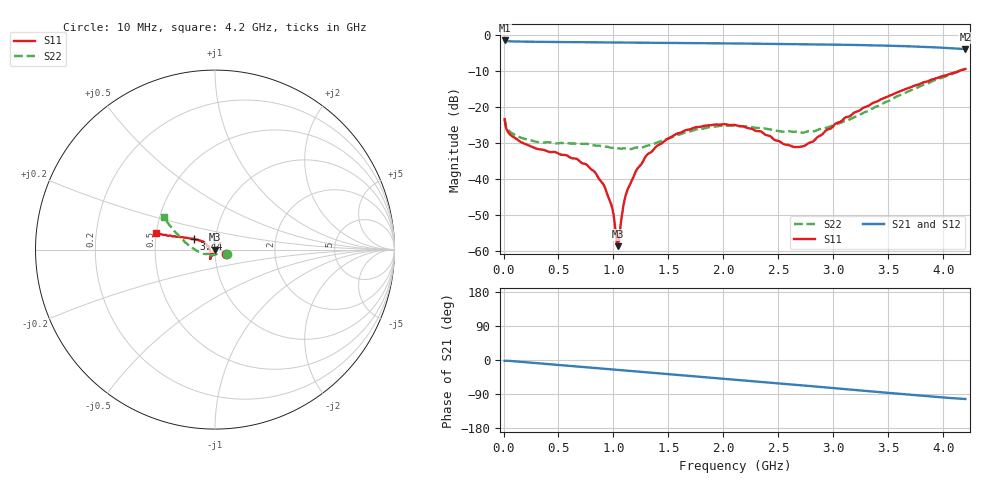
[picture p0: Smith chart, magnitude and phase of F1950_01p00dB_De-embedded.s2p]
! Integrated Device Technology
! Corporate Headquarters
! 6024 Silver Creek Valley Road
! San Jose, CA 95138  USA
! Phone:  1-408-284-8200
! Toll Free:  1-800-223-1366
! Webpage:  http://www.idt.com/
! Timing and RF Division
! 515 Groton Road, Suite 102
! Westford, MA 01886-6024
! Device:  F1950
! Description: 7-bit 0.25 dB Digital Step Attenuator
! Frequency:  150.0 -  4000.00 MHz
! Package:  4x4 mm Thin QFN Plastic Package: 24 pin
! Ports:  2 RF, 12 DC
!  Pin  1  = D0
!  Pin  2  = VDD
!  Pin  3  = Vmode
!  Pin  4  = GND
!  Pin  5  = RF1  =  Port 1
!  Pin  6  = GND
!  Pin  7  = GND
!  Pin  8  = GND
!  Pin  9  = GND
!  Pin 10  = GND
!  Pin 11  = GND
!  Pin 12  = GND
!  Pin 13  = GND
!  Pin 14  = RF2  =  Port 2
!  Pin 15  = GND
!  Pin 16  = LE
!  Pin 17  = CLK
!  Pin 18  = DATE
!  Pin 19  = D6
!  Pin 20  = D5
!  Pin 21  = D4
!  Pin 22  = D3
!  Pin 23  = D2
!  Pin 24  = D1
! State:  4
! Atten State:  1.00 dB
! Voltage:  +5.00 Volts
! Current:  Not Measured mA
! Data:  The device was measured on a the F195X evaluation board which has
!  individual transmission lines to the RF pins.  Data was collected
!  using a calibrated network analyzer.  The evaluation board was
!  de-embedded using a TRL calibration technique.
!  The reference plane is the edge of the package pin.
! Misc:  Board 2019
!  Action Tracker AT0250
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# GHz S dB R 50
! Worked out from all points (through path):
!   420 points, 10 MHz to 4.2 GHz, reference 50 ohm
!   highest |S21| = -1.47 dB at 10 MHz (marker M1); lowest = -3.9 dB at 4.2 GHz (marker M2)
!   group delay of S21, straight-line fit = 68.1 ps
!   lowest |S11| = -58.6 dB at 1.04 GHz (marker M3), VSWR 1.00, Z = 49.9 + j0.0154 ohm
!   |S11| at or under -10 dB: start of sweep to 4.136 GHz
!   |S22| runs from -31.6 to -9.4 dB; largest |S21 - S12| = 0.001
!   S11 on the Smith chart (normalised r, x): 10 MHz: 1.13, -0.06; 3.44 GHz: 0.79, +0.09; 4.2 GHz: 0.50, +0.10
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0.01  -23.35 -21.6  -1.47 -2.2  -1.47 -2.2  -23.08 -21.1
0.06  -27.63 -13.8  -1.71 -2.5  -1.71 -2.5  -26.86 -15.3
0.18  -30.02 -2.6  -1.80 -5.3  -1.80 -5.3  -28.71 -11.2
0.71  -35.49 50.1  -1.95 -18.2  -1.95 -18.2  -30.23 -12.9
0.82  -37.76 55.5  -1.97 -20.8  -1.97 -20.8  -30.64 -20.3
0.91  -41.57 65.0  -1.99 -23.0  -1.99 -23.0  -30.90 -29.2
0.98  -47.09 70.7  -2.01 -24.7  -2.01 -24.7  -31.31 -38.2
1.02  -54.81 108.9  -2.02 -25.7  -2.02 -25.7  -31.34 -44.3
1.04  -58.64 172.4  -2.02 -26.1  -2.02 -26.2  -31.47 -47.8
1.06  -54.00 -148.9  -2.03 -26.6  -2.03 -26.6  -31.52 -51.0
1.1  -45.91 -140.4  -2.03 -27.6  -2.03 -27.6  -31.46 -57.1
1.14  -42.11 -127.5  -2.04 -28.6  -2.04 -28.6  -31.60 -64.1
1.29  -33.85 -122.7  -2.08 -32.2  -2.07 -32.2  -30.92 -90.4
1.41  -30.48 -119.8  -2.11 -35.1  -2.11 -35.1  -29.70 -108.7
1.74  -25.63 -117.7  -2.20 -43.1  -2.19 -43.2  -26.28 -139.6
2.11  -25.00 -118.6  -2.31 -52.1  -2.31 -52.2  -25.21 -154.1
2.64  -31.05 -163.3  -2.47 -65.0  -2.47 -65.1  -26.88 -151.6
2.81  -29.61 163.3  -2.54 -69.3  -2.53 -69.3  -26.75 -150.0
3.11  -22.87 147.4  -2.67 -76.9  -2.67 -77.0  -23.78 -158.8
3.44  -17.73 153.2  -2.89 -85.3  -2.88 -85.4  -19.20 -179.7
3.51  -16.83 154.7  -2.94 -87.1  -2.93 -87.1  -18.18 176.5
4.2  -9.40 164.4  -3.88 -102.9  -3.87 -103.0  -9.40 147.7
